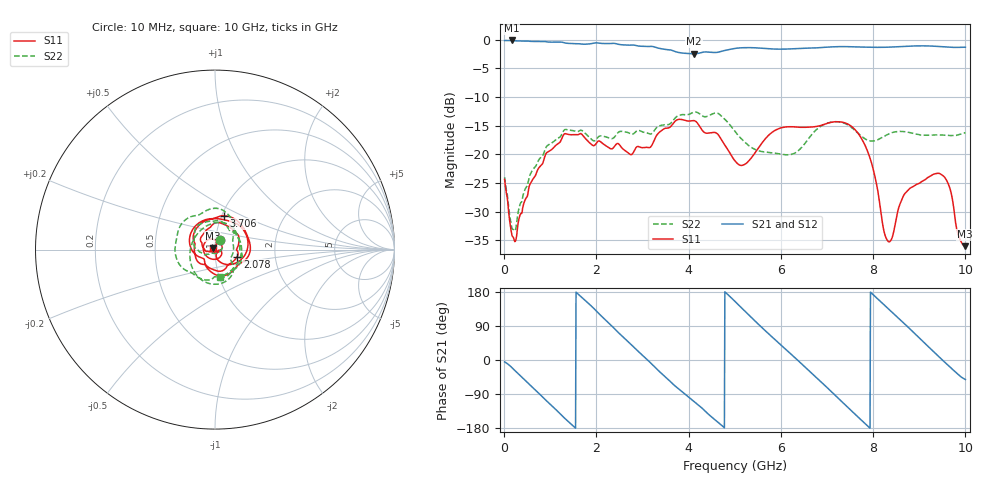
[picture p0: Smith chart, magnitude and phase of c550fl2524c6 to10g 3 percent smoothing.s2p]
!Agilent Technologies,N5234A,MY52241123,A.10.00.00
!Agilent N5234A: A.10.00.00
!Date: Monday, May 06, 2019 14:09:59
!Correction: S11(Full 2 Port(1,2))
!S21(Full 2 Port(1,2))
!S12(Full 2 Port(1,2))
!S22(Full 2 Port(1,2))
!S2P File: Measurements: S11, S21, S12, S22:
# Hz S  dB  R 50
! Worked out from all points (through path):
!   1001 points, 10 MHz to 10 GHz, reference 50 ohm
!   highest |S21| = -0.11 dB at 159.8 MHz (marker M1); lowest = -2.4 dB at 4.116 GHz (marker M2)
!   group delay of S21, straight-line fit = 314 ps
!   lowest |S11| = -36.0 dB at 9.99 GHz (marker M3), VSWR 1.03, Z = 48.7 + j0.907 ohm
!   |S11| at or under -10 dB: start of sweep to end of sweep
!   |S22| runs from -33.3 to -12.6 dB; largest |S21 - S12| = 0.0019
!   S11 on the Smith chart (normalised r, x): 10 MHz: 1.05, +0.11; 2.078 GHz: 1.28, -0.10; 3.706 GHz: 1.03, +0.40; 10 GHz: 0.97, +0.02
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1e7  -24.35 62.7  -0.13 -5.0  -0.11 -4.9  -23.96 61.5
1.5985e8  -33.69 -52.8  -0.11 -19.2  -0.11 -19.1  -32.51 -45.8
8.4916e8  -21.27 151.6  -0.28 -99.3  -0.28 -99.3  -20.01 179.0
1.27873e9  -16.71 91.6  -0.46 -149.8  -0.45 -149.8  -16.01 134.8
1.67833e9  -16.43 28.1  -0.74 165.4  -0.74 165.4  -15.79 81.2
2.07793e9  -17.70 -17.9  -0.60 119.5  -0.60 119.5  -16.76 36.3
2.4076e9  -18.42 -59.6  -0.64 80.6  -0.64 80.6  -16.80 -3.9
2.81719e9  -19.40 -129.9  -0.92 33.3  -0.92 33.3  -16.31 -55.0
3.34666e9  -16.27 135.9  -1.46 -28.3  -1.46 -28.3  -15.06 -106.5
3.7063e9  -14.21 75.1  -2.05 -68.5  -2.05 -68.6  -13.64 -150.5
4.11589e9  -14.10 2.3  -2.44 -109.5  -2.44 -109.5  -12.59 144.9
5.005e9  -21.12 -131.3  -1.50 154.6  -1.50 154.6  -15.97 47.7
5.69431e9  -16.97 170.0  -1.53 73.5  -1.53 73.5  -19.61 9.4
6.22378e9  -15.16 106.9  -1.58 15.1  -1.58 15.1  -19.99 -30.1
6.67333e9  -15.21 73.7  -1.43 -35.6  -1.43 -35.6  -16.49 -46.5
7.34266e9  -14.39 18.5  -1.18 -112.4  -1.18 -112.4  -14.45 -105.0
7.84216e9  -18.72 -46.1  -1.28 -169.7  -1.28 -169.8  -17.36 175.4
8.34166e9  -35.23 -34.6  -1.28 134.2  -1.28 134.1  -16.41 85.5
8.81119e9  -25.83 -64.0  -1.09 80.5  -1.09 80.4  -16.21 43.1
9.29071e9  -23.52 169.6  -1.10 24.3  -1.10 24.2  -16.62 17.0
9.99001e9  -35.99 144.1  -1.29 -50.8  -1.29 -50.9  -16.21 -79.2
1e10  -35.98 147.7  -1.29 -51.4  -1.29 -51.5  -16.19 -80.0
